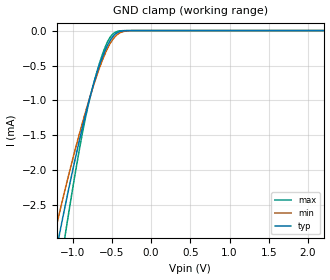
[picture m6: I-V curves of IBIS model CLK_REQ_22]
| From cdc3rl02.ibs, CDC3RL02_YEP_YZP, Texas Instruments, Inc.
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[Model]   CLK_REQ_22
Model_type  Input
Vinl=0.5
Vinh=1.3
| variable   typ   min   max
C_comp   1.86pF   1.32pF   2.07pF
[Temperature Range]   40   100   -40
| Ambient temperature   25   85   -40
[Voltage range]   2.2   2   2.4
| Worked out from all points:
|   GND clamp passes 1 mA (typ) near -0.79 V on its own axis
[GND Clamp]
| CLK_REQ_22
|   Voltage   I(typ)   I(min)   I(max)
-2.2V     -9.667mA   -8.323mA   -12.08mA
-1.22V    -3.213mA   -2.859mA   -3.851mA
-1.17V    -2.927mA   -2.619mA   -3.477mA
-1.1V     -2.538mA   -2.293mA   -2.966mA
-1.075V   -2.402mA   -2.178mA   -2.788mA
-870mV    -1.363mA   -1.301mA   -1.438mA
-760mV    -875.4uA   -881.2uA   -880.8uA
-600mV    -324.4uA   -367uA     -279.4uA
-530mV    -159.1uA   -202uA     -111.1uA
-460mV    -54.21uA   -88.3uA    -27.41uA
-250mV    -230.4nA   -1.251uA   -15.48nA
2.2V      103.7pA    3.403nA    49.54pA
